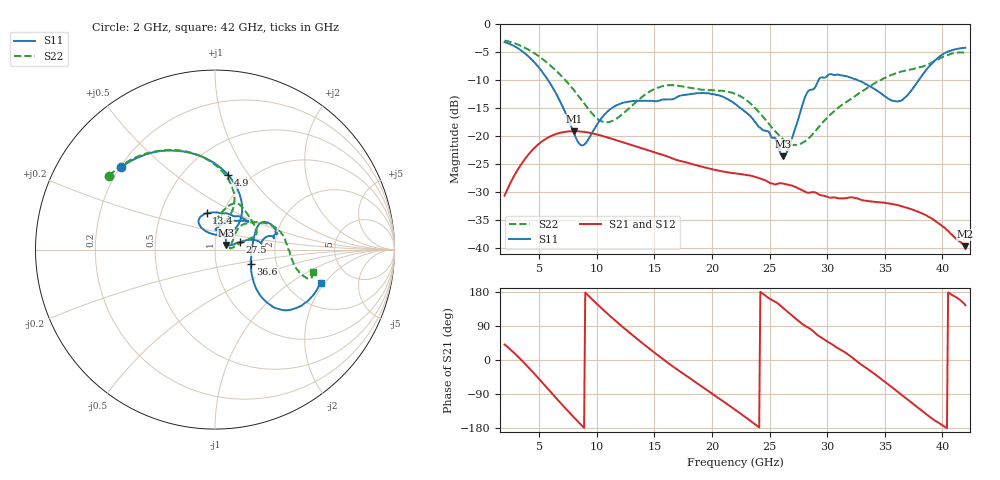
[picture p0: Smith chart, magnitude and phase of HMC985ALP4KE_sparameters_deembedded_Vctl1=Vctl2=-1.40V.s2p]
!s2p File: Measurements: S11, S21, S12, S22
# GHz S dB R 50.0
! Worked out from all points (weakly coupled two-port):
!   401 points, 2 GHz to 42 GHz, reference 50 ohm
!   highest |S21| = -19.11 dB at 8 GHz (marker M1); lowest = -39.7 dB at 42 GHz (marker M2)
!   lowest |S11| = -23.6 dB at 26.2 GHz (marker M3), VSWR 1.14, Z = 56.4 + j2.91 ohm
!   |S11| at or under -10 dB: 5.78 GHz to 29.25 GHz (23.47 GHz wide, 134 % of centre); 32.67 GHz to 37.94 GHz (5.269 GHz wide, 14.9 % of centre)
!   |S22| runs from -21.6 to -2.9 dB; largest |S21 - S12| = 0.00013
!   S11 on the Smith chart (normalised r, x): 2 GHz: 0.20, +0.36; 4.9 GHz: 0.80, +0.81; 13.4 GHz: 0.84, +0.36; 27.5 GHz: 1.31, +0.11; 36.6 GHz: 1.47, -0.25; 42 GHz: 3.06, -1.84
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2  -3.15 138.5  -30.66 40.9  -30.67 41.0  -2.87 145.1
3.4  -4.62 110.7  -25.16 1.6  -25.17 1.7  -3.83 122.0
4.9  -7.52 79.8  -21.51 -46.9  -21.52 -47.0  -5.59 98.4
6.2  -11.40 55.9  -19.83 -91.3  -19.84 -91.3  -7.76 80.7
8  -19.41 54.1  -19.11 -150.9  -19.12 -150.9  -11.72 66.5
8.7  -21.67 81.5  -19.19 -172.8  -19.20 -172.8  -13.60 66.5
10.8  -15.86 122.2  -20.15 125.7  -20.15 125.7  -17.52 85.2
13.4  -13.68 103.0  -21.83 58.3  -21.83 58.3  -13.89 81.5
15.4  -13.65 76.5  -23.16 10.5  -23.16 10.5  -11.24 68.7
18.9  -12.32 41.0  -25.35 -65.3  -25.36 -65.3  -11.61 42.3
22  -14.21 55.6  -26.66 -130.8  -26.67 -130.8  -12.42 19.6
24.5  -18.97 88.9  -27.81 173.0  -27.82 173.0  -16.68 14.0
26.2  -23.59 22.9  -28.51 136.6  -28.51 136.6  -20.61 5.0
27.5  -16.89 16.5  -29.34 103.3  -29.33 103.3  -21.49 7.5
28.2  -12.46 12.3  -30.07 88.0  -30.08 87.8  -20.74 16.2
28.7  -11.66 7.7  -30.03 78.2  -30.04 78.1  -19.74 23.0
31.1  -9.07 19.4  -31.14 28.3  -31.14 28.4  -14.69 42.9
33.3  -10.60 30.3  -31.55 -19.1  -31.55 -19.0  -11.63 35.3
35.4  -13.39 9.7  -32.06 -66.6  -32.09 -66.6  -9.22 22.6
36.6  -13.36 -21.7  -32.63 -95.2  -32.65 -95.2  -8.39 13.9
39.6  -6.03 -42.2  -35.51 -164.5  -35.48 -164.5  -6.29 -15.0
42  -4.16 -17.4  -39.70 144.3  -39.67 144.3  -5.08 -12.7
